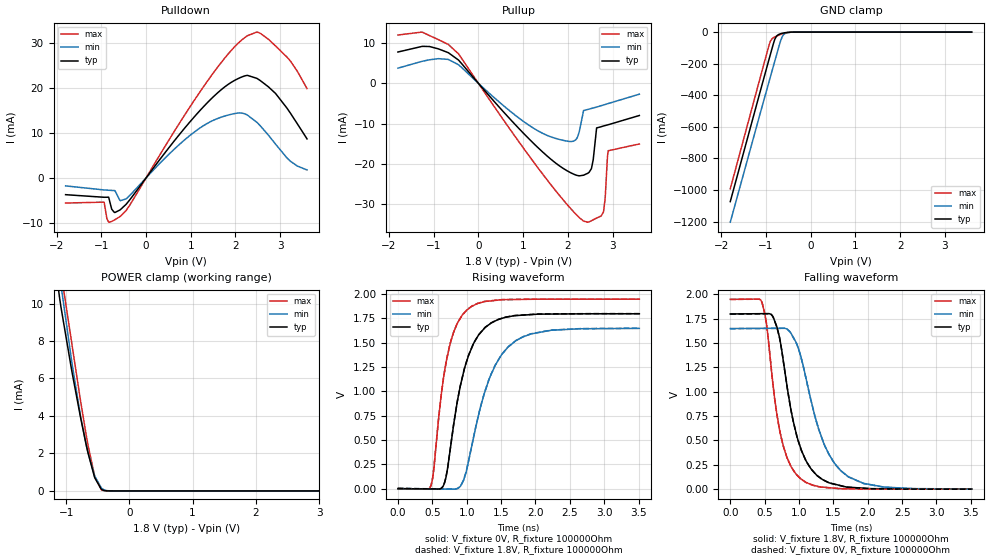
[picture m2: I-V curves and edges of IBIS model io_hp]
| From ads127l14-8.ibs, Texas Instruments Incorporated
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|   io_hp Model
[Model]   io_hp
Model_type   I/O
Polarity   Non-Inverting
Enable   Active-Low
Vinl = 0.54
Vinh = 1.26
Vmeas = 0.9
Vref = 0
Cref = 2pF
Rref = 100000
|   typ   min   max
C_comp   0.609pF   0.629pF   0.591pF
[Voltage Range]   1.8   1.65   1.95
[Temperature Range]   27   125   -40
[Pullup Reference]   1.8   1.65   1.95
[Pulldown Reference]   0   0   0
[Power Clamp Reference]   1.8   1.65   1.95
[GND Clamp Reference]   0   0   0
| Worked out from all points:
|   slope of the pulldown table from 0 to 0.27 V, typ, clamps not added: 75.1 ohm
|   slope of the pullup table from 0 to 0.27 V, typ, clamps not added: 77.9 ohm
|   GND clamp passes 1 mA (typ) near -0.47 V on its own axis
|   POWER clamp passes 1 mA (typ) near -0.57 V on its own axis
|   falling waveform, V_fixture 1.8V, R_fixture 100000Ohm: 20-80 % time 313ps typ, 417ps min, 245ps max; typ from 1.8 V to 0.001 V
|   rising waveform, V_fixture 0V, R_fixture 100000Ohm: 20-80 % time 316ps typ, 417ps min, 241ps max; typ from 0 V to 1.8 V
|   rising waveform, V_fixture 1.8V, R_fixture 100000Ohm: 20-80 % time 316ps typ, 416ps min, 240ps max; typ from 0.001 V to 1.8 V
|   falling waveform, V_fixture 0V, R_fixture 100000Ohm: 20-80 % time 313ps typ, 417ps min, 245ps max; typ from 1.8 V to 0 V
[Pulldown]
|   Voltage   I(typ)   I(min)   I(max)
-1.8V     -3.724mA   -1.772mA   -5.583mA
-941.4mV  -4.299mA   -2.672mA   -5.381mA
-838.8mV  -4.272mA   -2.741mA   -9.781mA
-709.2mV  -7.669mA   -2.804mA   -9.344mA
-574.2mV  -7.044mA   -5.058mA   -8.515mA
1.219V    15.11mA    11.18mA    19.3mA
1.775V    20.33mA    13.79mA    26.79mA
2.266V    22.78mA    13.97mA    31.59mA
2.477V    22.12mA    12.36mA    32.39mA
2.741V    20.19mA    9.434mA    30.76mA
3.233V    14.31mA    3.676mA    25.91mA
3.6V      8.67mA     1.764mA    19.85mA
[GND Clamp]
|   Voltage   I(typ)   I(min)   I(max)
-1.8V     -1.073A    -1.203A    -991.6mA
-1.071V   -314.6mA   -454.1mA   -226.3mA
-909mV    -148.1mA   -289.9mA   -62.57mA
-865.8mV  -104.2mA   -246.2mA   -42.09mA
-811.8mV  -51.93mA   -191.7mA   -31.97mA
-768.6mV  -27.22mA   -148.2mA   -26.46mA
-671.4mV  -10.31mA   -52.75mA   -15.22mA
-633.6mV  -7.434mA   -27.57mA   -11.39mA
-590.4mV  -4.838mA   -11.77mA   -7.591mA
-536.4mV  -2.477mA   -3.932mA   -3.947mA
-369mV    -68.86uA   -116.7uA   -98.27uA
3.6V      0A         0A         0A
[Pullup]
|   Voltage   I(typ)   I(min)   I(max)
-1.8V     7.792mA    3.775mA    12.03mA
-1.265V   9.179mA    5.458mA    12.75mA
-444.6mV  5.786mA    4.621mA    7.335mA
1.597V    -18.65mA   -13.21mA   -24.87mA
2.18V     -22.82mA   -14.02mA   -32.54mA
2.353V    -22.85mA   -6.766mA   -34.28mA
2.531V    -21.1mA    -6.243mA   -34.18mA
2.644V    -11.1mA    -5.902mA   -33.52mA
2.795V    -10.62mA   -5.391mA   -32.04mA
2.833V    -10.51mA   -5.263mA   -28.84mA
2.903V    -10.3mA    -5.028mA   -16.77mA
3.6V      -8mA       -2.698mA   -15.08mA
[POWER Clamp]
|   Voltage   I(typ)   I(min)   I(max)
-1.8V     31.21mA    30.7mA     34.75mA
-1.103V   10.28mA    11.52mA    12.12mA
-1.082V   9.797mA    10.98mA    11.66mA
-914.4mV  6.469mA    6.968mA    7.947mA
-774mV    3.948mA    4.022mA    4.833mA
-687.6mV  2.529mA    2.527mA    3.066mA
-655.2mV  2.04mA     2.046mA    2.454mA
-547.2mV  695.3uA    782.9uA    771uA
-439.2mV  77.92uA    141.2uA    59.87uA
-374.4mV  11.15uA    32.03uA    6.079uA
-261mV    174.7nA    1.497uA    51.88nA
3.6V      0A         0A         0A
[Ramp]
R_load = 100000
|   typ   min   max
dV/dt_r   1.07917/3.12946e-10   0.989044/4.12093e-10   1.16929/2.40102e-10
dV/dt_f   1.0792/3.10526e-10   0.989082/4.14531e-10   1.1693/2.42665e-10
[Falling Waveform]
V_fixture = 1.8V
V_fixture_min = 1.65V
V_fixture_max = 1.95V
R_fixture = 100000Ohm
C_fixture = 0F
|   Time   V(typ)   V(min)   V(max)
0s        1.8V       1.65V      1.95V
459.5ps   1.803V     1.652V     1.921V
525.2ps   1.803V     1.652V     1.71V
617.6ps   1.776V     1.653V     1.101V
767.7ps   1.338V     1.654V     453.5mV
885.5ps   805.4mV    1.599V     230.3mV
1.022ns   426.1mV    1.374V     108.3mV
1.356ns   94.24mV    479.7mV    20.03mV
1.709ns   20.95mV    132mV      4.583mV
3.512ns   1.43mV     1.714mV    1.195mV
[Rising Waveform]
V_fixture = 0V
V_fixture_min = 0V
V_fixture_max = 0V
R_fixture = 100000Ohm
C_fixture = 0F
|   Time   V(typ)   V(min)   V(max)
0s        5.563nV    56.21nV    55.5nV
477.9ps   -3.564mV   -3.169mV   26.38mV
521.8ps   -3.892mV   -3.461mV   201.7mV
638.1ps   5.22mV     -4.232mV   1.008V
711.5ps   164.5mV    -4.718mV   1.338V
873.5ps   933mV      2.05mV     1.712V
1.001ns   1.311V     196.1mV    1.836V
1.322ns   1.686V     1.116V     1.929V
1.709ns   1.78V      1.518V     1.945V
3.512ns   1.799V     1.648V     1.949V
[Rising Waveform]
V_fixture = 1.8V
V_fixture_min = 1.65V
V_fixture_max = 1.95V
R_fixture = 100000Ohm
C_fixture = 0F
|   Time   V(typ)   V(min)   V(max)
0s        1.332mV    1.528mV    1.161mV
477.9ps   -2.208mV   -1.603mV   27.61mV
521.8ps   -2.534mV   -1.891mV   203mV
638.1ps   6.634mV    -2.653mV   1.01V
711.5ps   166.1mV    -3.133mV   1.34V
873.5ps   934.8mV    3.718mV    1.713V
1.001ns   1.313V     198.2mV    1.837V
1.322ns   1.687V     1.118V     1.93V
1.709ns   1.781V     1.52V      1.947V
3.512ns   1.8V       1.65V      1.95V
[Falling Waveform]
|Gnd
V_fixture = 0V
V_fixture_min = 0V
V_fixture_max = 0V
R_fixture = 100000Ohm
C_fixture = 0F
|   Time   V(typ)   V(min)   V(max)
0s        1.799V     1.648V     1.949V
459.5ps   1.802V     1.651V     1.92V
525.2ps   1.802V     1.651V     1.708V
617.6ps   1.775V     1.651V     1.1V
767.7ps   1.336V     1.652V     452.1mV
885.5ps   803.5mV    1.597V     229.1mV
1.022ns   424.5mV    1.372V     107.1mV
1.356ns   92.84mV    477.5mV    18.86mV
1.709ns   19.6mV     130.3mV    3.421mV
3.512ns   98.34uV    186.1uV    34.58uV
